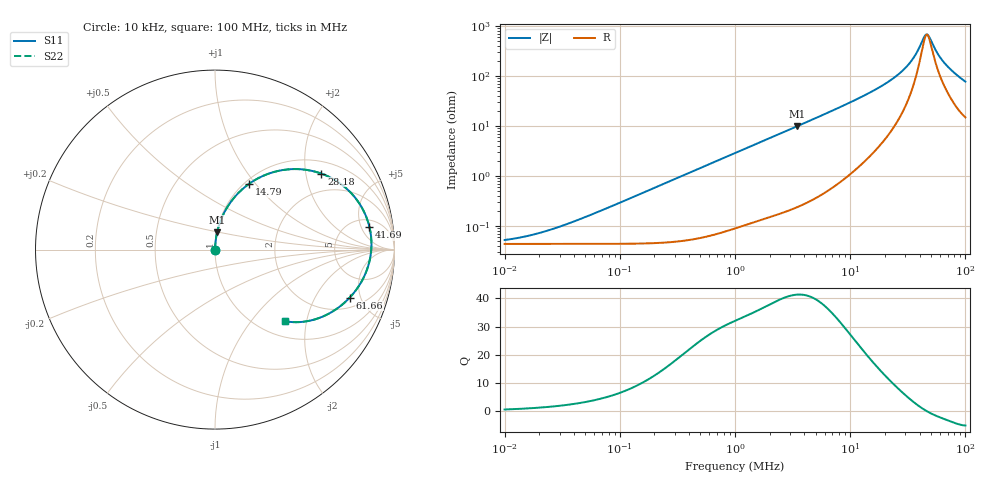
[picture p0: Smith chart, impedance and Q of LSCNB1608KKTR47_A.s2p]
! LSCNB1608KKTR47_A  S-PARAMETER MODEL  ( Standard Model )
! Model Generated by TAIYO YUDEN Corporation (http://www.ty-top.com)
! Version 2.0
! TAIYO YUDEN Control No. 171005
! Copyright(c) 2017 TAIYO YUDEN CO.,LTD. All Rights Reserved.
! Product Description (link to TY-COMPAS)
! https://ds.yuden.co.jp/TYCOMPAS/or/detail?pn=LSCNB1608KKTR47MA&u=M
! Products Name : Inductors
! Characteristics :
!  Inductance : 0.47 [uH] , SRF(min) : - [Hz] , DC Resistance(max) : 55 [mOhm]
!  Rated Current : Saturation  2.4 [A] (dL = 30 [%]), Temp Rise  2.0 [A] (dT = 40 [degC])
!  Case Size : 1.6 x 0.8 / 0.063 x 0.031 [mm/inch] , Thickness : 1.0 / 0.039 [mm/inch]
!  (Conditions: Temperature = 25 [degC] , DC Bias Current = 0 [A])
! External Node Assignments :
!  1  o---GGG---o  2
! GND o---------o GND
! Frequency Range : 10kHz  -  100MHz  [ 402 STEP ]
# MHz S RI R 50
! Freq[MHz].  S11 Real  S11 Imag  S21 Real  S21 Imag  S12 Real  S12 Imag  S22 Real  S22 Imag
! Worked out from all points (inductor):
!   401 points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, 10 kHz to 100 MHz, reference 50 ohm
!   read as one part in series: L = 460 nH near 45.71 kHz
!   highest Q = 41.3 at 3.467 MHz (marker M1), where L = 453 nH
!   self-resonance near 46.5 MHz
!   S11 on the Smith chart (normalised r, x): 10 kHz: 1.00, +0.00; 14.79 MHz: 1.05, +0.92; 28.18 MHz: 1.36, +2.46; 41.69 MHz: 6.94, +7.14; 61.66 MHz: 2.73, -4.00; 100 MHz: 1.30, -1.51
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0.01  0.00044 0.000289  0.9996 -0.000289  0.9996 -0.000289  0.00044 0.000289
0.020417  0.00044 0.00059  0.9996 -0.00059  0.9996 -0.00059  0.00044 0.00059
0.046774  0.000442 0.00135  0.9996 -0.00135  0.9996 -0.00135  0.000442 0.00135
0.218776  0.000501 0.00633  0.9995 -0.00633  0.9995 -0.00633  0.000501 0.00633
1  0.00172 0.0287  0.9983 -0.0287  0.9983 -0.0287  0.00172 0.0287
3.467369  0.012 0.0973  0.988 -0.0973  0.988 -0.0973  0.012 0.0973
4.677351  0.0206 0.1303  0.9794 -0.1303  0.9794 -0.1303  0.0206 0.1303
9.120108  0.074 0.2452  0.926 -0.2452  0.926 -0.2452  0.074 0.2452
14.79108  0.1892 0.3658  0.8108 -0.3658  0.8108 -0.3658  0.1892 0.3658
18.19701  0.2804 0.4161  0.7196 -0.4161  0.7196 -0.4161  0.2804 0.4161
21.87762  0.3922 0.4454  0.6078 -0.4454  0.6078 -0.4454  0.3922 0.4454
28.18383  0.5931 0.4232  0.4069 -0.4232  0.4069 -0.4232  0.5931 0.4232
34.67368  0.7647 0.3083  0.2353 -0.3083  0.2353 -0.3083  0.7647 0.3083
38.01894  0.8235 0.2244  0.1765 -0.2244  0.1765 -0.2244  0.8235 0.2244
41.68694  0.8607 0.1253  0.1393 -0.1253  0.1393 -0.1253  0.8607 0.1253
44.66836  0.8715 0.0461  0.1285 -0.0461  0.1285 -0.0461  0.8715 0.0461
46.77351  0.8701 -0.00677  0.1299 0.00677  0.1299 0.00677  0.8701 -0.00677
48.97788  0.8622 -0.0582  0.1378 0.0582  0.1378 0.0582  0.8622 -0.0582
56.23413  0.8064 -0.1949  0.1936 0.1949  0.1936 0.1949  0.8064 -0.1949
61.6595  0.7508 -0.2671  0.2492 0.2671  0.2492 0.2671  0.7508 -0.2671
77.62471  0.5812 -0.3807  0.4188 0.3807  0.4188 0.3807  0.5812 -0.3807
100  0.3912 -0.3993  0.6088 0.3993  0.6088 0.3993  0.3912 -0.3993
